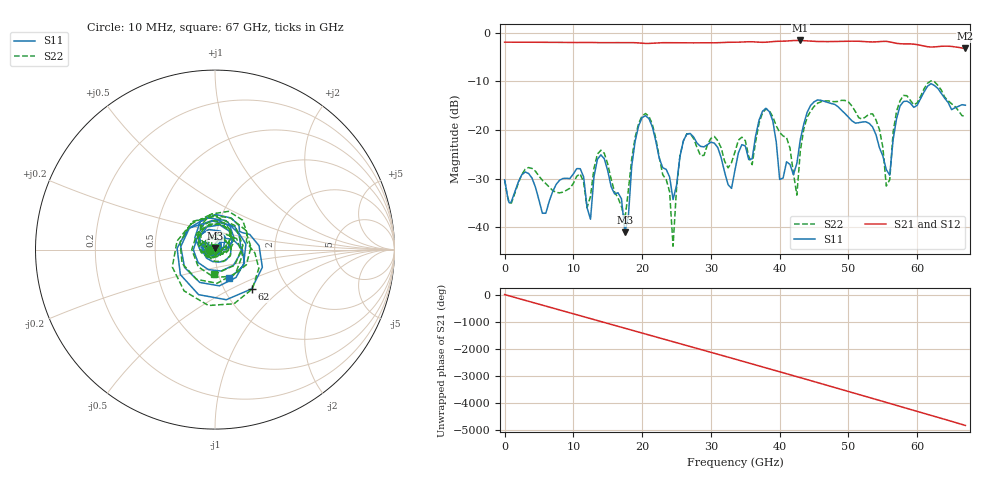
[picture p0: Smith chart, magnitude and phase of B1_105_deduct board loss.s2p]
!Keysight Technologies,N5247B,MY61255065,A.16.20.04
!Date: Sunday, September 03, 2023 21:47:20
!Correction: S11(C  2-Port  )
!S21(C  2-Port  )
!S12(C  2-Port  )
!S22(C  2-Port  )
!S2P File: Measurements: S11, S21, S12, S22:
!Deduct Board Loss
# Hz S  dB  R 50
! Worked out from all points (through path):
!   142 points, 10 MHz to 67 GHz, reference 50 ohm
!   highest |S21| = -1.59 dB at 43 GHz (marker M1); lowest = -3.2 dB at 67 GHz (marker M2)
!   lowest |S11| = -41.1 dB at 17.5 GHz (marker M3), VSWR 1.02, Z = 50 + j0.883 ohm
!   |S11| at or under -10 dB: start of sweep to end of sweep
!   |S22| runs from -43.9 to -9.9 dB; largest |S21 - S12| = 0.0033
!   S11 on the Smith chart (normalised r, x): 10 MHz: 0.94, -0.00; 62 GHz: 1.33, -0.64; 67 GHz: 1.11, -0.37
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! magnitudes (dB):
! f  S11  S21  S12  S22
! 10 MHz  -30.3  -1.9  -1.9  -30.3
! 11.5 GHz  -29.7  -2.0  -2.0  -30.8
! 12.5 GHz  -38.4  -2.0  -2.0  -33.7
! 14.5 GHz  -25.9  -2.0  -2.0  -24.8
! 17.5 GHz  -41.1  -2.0  -2.0  -38.5
! 20 GHz  -17.5  -2.2  -2.2  -17.1
! 22.5 GHz  -25.9  -2.1  -2.1  -25.7
! 24.5 GHz  -34.3  -2.1  -2.1  -43.9
! 26.5 GHz  -20.9  -2.1  -2.1  -20.8
! 33 GHz  -32.0  -2.0  -2.0  -26.7
! 34 GHz  -24.7  -1.9  -1.9  -22.1
! 36 GHz  -25.9  -1.9  -1.9  -27.1
! 38.5 GHz  -16.2  -1.9  -1.9  -16.0
! 40 GHz  -30.2  -1.8  -1.8  -20.5
! 42.5 GHz  -26.9  -1.6  -1.6  -33.4
! 43 GHz  -22.0  -1.6  -1.6  -24.3
! 45 GHz  -14.2  -1.8  -1.8  -15.2
! 53.5 GHz  -19.4  -1.9  -1.9  -16.7
! 56 GHz  -29.3  -1.9  -1.9  -30.3
! 57.5 GHz  -15.1  -2.3  -2.3  -14.0
! 62 GHz  -10.5  -2.9  -2.9  -9.9
! 67 GHz  -14.9  -3.2  -3.2  -17.2
